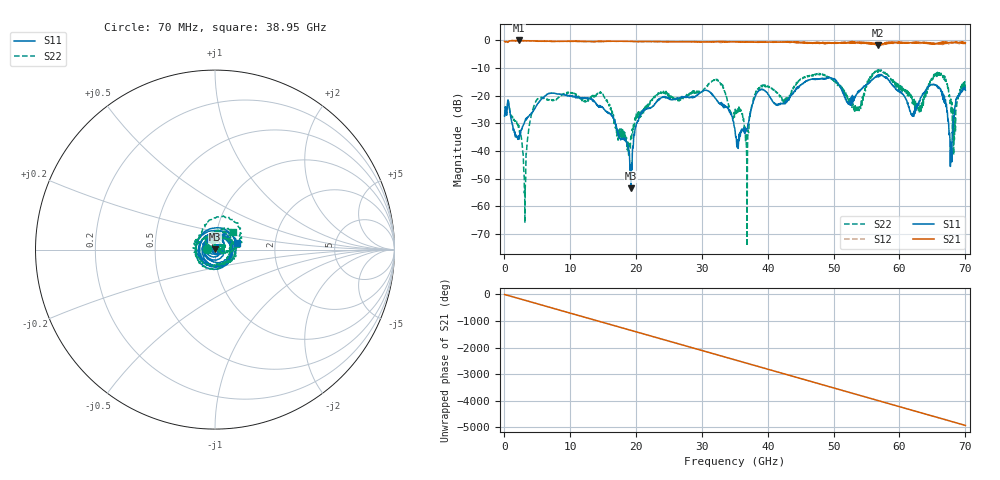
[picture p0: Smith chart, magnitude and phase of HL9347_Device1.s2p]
! 4/22/2025 2:28:54 PM
! H:\PROTOTYPE_DATA\DC_FEEDER_67GHZ\PROTO1.S2P
! CHANNEL.1
! TR.MEASUREMENT
! CORRECTED.DATA
# GHZ S RI R 50.0
! FREQ.GHZ  S11RE  S11IM  S21RE  S21IM  S12RE  S12IM  S22RE  S22IM
!; PortSelection: Port_12
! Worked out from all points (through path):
!   1999 points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, 70 MHz to 70 GHz, reference 50 ohm
!   highest |S21| = -0.08 dB at 2.205 GHz (marker M1); lowest = -1.9 dB at 56.7 GHz (marker M2)
!   group delay of S21, straight-line fit = 195 ps
!   lowest |S11| = -53.4 dB at 19.25 GHz (marker M3), VSWR 1.00, Z = 50.1 + j0.196 ohm
!   |S11| at or under -10 dB: start of sweep to end of sweep
!   |S22| runs from -74.4 to -10.7 dB; largest |S21 - S12| = 0.12
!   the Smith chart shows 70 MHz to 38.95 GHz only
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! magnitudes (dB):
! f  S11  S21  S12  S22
! 70 MHz  -27.4  -0.4  -0.4  -27.4
! 2.205 GHz  -34.4  -0.1  -0.1  -30.7
! 3.115 GHz  -29.4  -0.1  -0.1  -53.7
! 4.97 GHz  -23.4  -0.3  -0.3  -21.5
! 11.72 GHz  -20.8  -0.4  -0.3  -21.1
! 14.77 GHz  -24.2  -0.4  -0.4  -18.7
! 19.25 GHz  -53.4  -0.4  -0.4  -34.5
! 20.55 GHz  -27.9  -0.5  -0.5  -28.1
! 23.38 GHz  -21.5  -0.5  -0.5  -19.0
! 30.94 GHz  -18.2  -0.6  -0.6  -15.9
! 35.03 GHz  -32.4  -0.5  -0.6  -25.4
! 36.82 GHz  -32.1  -0.7  -0.6  -43.5
! 38.53 GHz  -18.5  -0.7  -0.8  -17.7
! 46.69 GHz  -14.1  -0.9  -1.0  -12.9
! 53.52 GHz  -19.4  -0.9  -0.7  -24.7
! 56.7 GHz  -13.1  -1.9  -1.6  -11.4
! 58.34 GHz  -14.5  -1.1  -0.9  -13.0
! 62.97 GHz  -22.2  -0.9  -1.1  -23.6
! 65.91 GHz  -16.8  -1.0  -1.0  -11.6
! 67.8 GHz  -36.8  -0.7  -1.0  -21.2
! 68.32 GHz  -27.1  -0.8  -0.9  -35.9
! 70 GHz  -18.1  -1.0  -1.0  -17.3
